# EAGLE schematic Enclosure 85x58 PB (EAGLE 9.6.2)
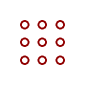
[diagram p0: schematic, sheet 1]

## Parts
U$1  PROTO-28X18  [PROTO-28X18]

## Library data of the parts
U$1 = digitalconcepts:PROTO-28X18: 28 x 18 Prototyping board to fit an 85 x 58 enclosure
